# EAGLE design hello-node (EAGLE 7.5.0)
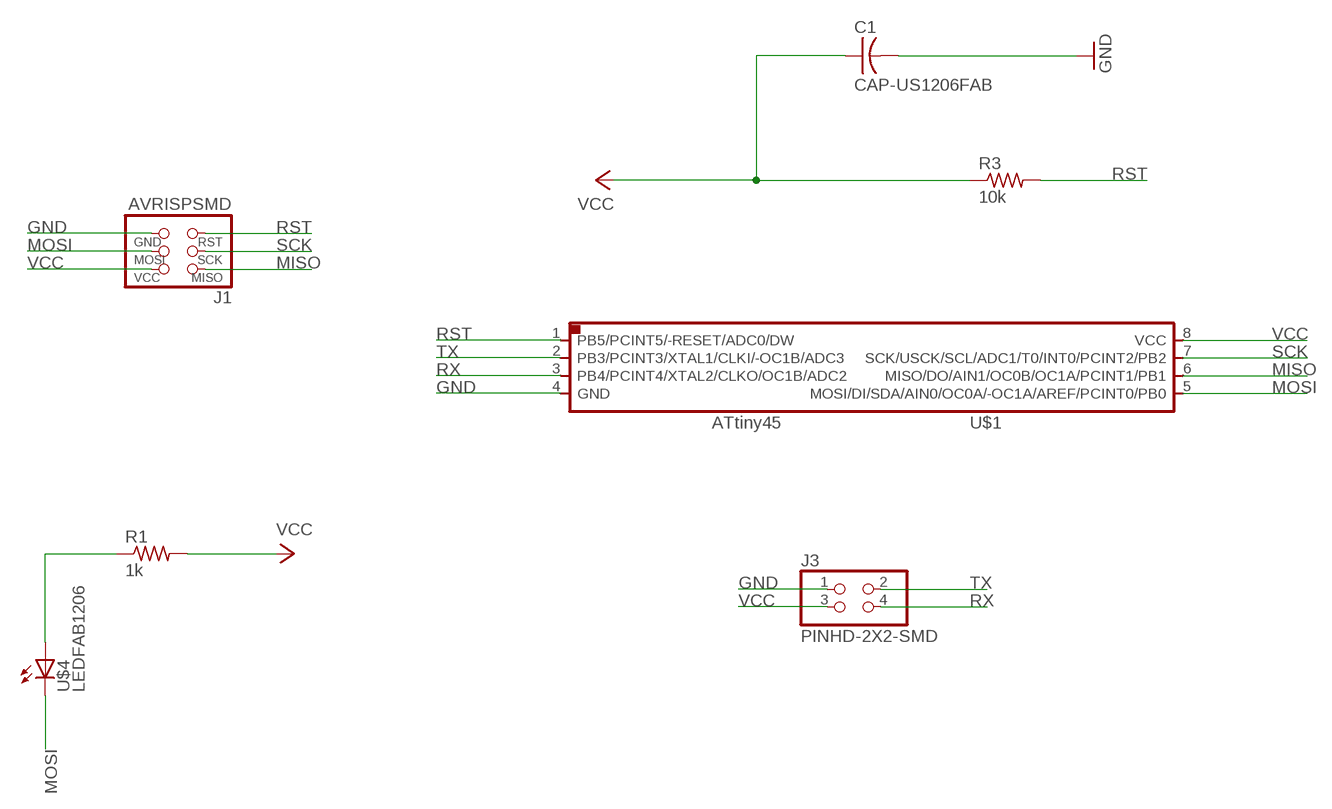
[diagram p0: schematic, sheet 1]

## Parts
C1  CAP-US1206FAB  [C1206FAB]
J1  AVRISPSMD  [2X03SMD]
J3  PINHD-2X2-SMD  [2X02SMD]
R1  1k  RES-US1206FAB  [R1206FAB]
R3  10k  RES-US1206FAB  [R1206FAB]
U$1  ATTINY45SI  [SOIC8]
U$4  LEDFAB1206  [LED1206FAB]

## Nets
GND: C1.2 J1.6(GND) J3.1 U$1.4(GND)
MISO: J1.1(MISO) U$1.6(MISO/DO/AIN1/OC0B/OC1A/PCINT1/PB1)
MOSI: J1.4(MOSI) U$1.5(MOSI/DI/SDA/AIN0/OC0A/-OC1A/AREF/PCINT0/PB0) U$4.2(C)
N$1: R1.1 U$4.1(A)
RST: J1.5(RST) R3.2 U$1.1(PB5/PCINT5/-RESET/ADC0/DW)
RX: J3.4 U$1.3(PB4/PCINT4/XTAL2/CLKO/OC1B/ADC2)
SCK: J1.3(SCK) U$1.7(SCK/USCK/SCL/ADC1/T0/INT0/PCINT2/PB2)
TX: J3.2 U$1.2(PB3/PCINT3/XTAL1/CLKI/-OC1B/ADC3)
VCC: C1.1 J1.2(VCC) J3.3 R1.2 R3.1 U$1.8(VCC)

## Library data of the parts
C1 = 01-fab:CAP-US
J1 = 01-fab:AVRISP
J3 = 01-fab:PINHD-2X2-SMD
R1 R3 = 01-fab:RES-US: Resistor (US Symbol)
U$1 = 01-fab:ATTINY45
U$4 = 01-fab:LED: LED

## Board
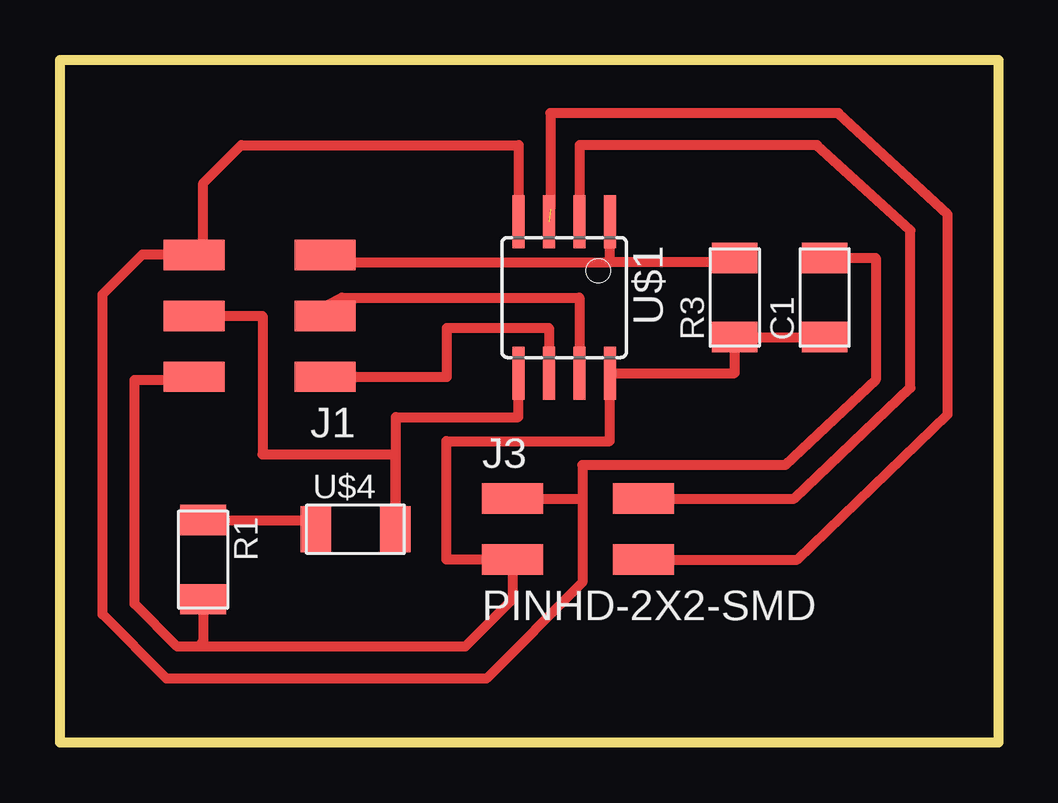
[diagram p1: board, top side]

Size 39.1 x 28.44 mm. Coordinates in mm from the lower left corner, seen from the top.
Outline: 0,0 39.1,0 39.1,28.44 0,28.44 0,0
Copper layers (1*16): Top 0.035mm / dielectric 1.5mm / Bottom 0.035mm
Design rules "default *": minimum track width 10mil, minimum drill 24mil, track to track 16mil, track to pad 16mil, pad to pad 16mil, via to via 16mil, smd to smd 16mil, copper to edge 40mil, drill to drill 8mil, minimum pad ring 10mil, minimum via ring 8mil, stop-mask expansion 4mil, vias tented up to drill 0mil, thermal gap 10mil
Milling: 4 lines

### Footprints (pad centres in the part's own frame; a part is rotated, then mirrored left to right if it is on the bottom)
C1206FAB = smd 1.27 x 1.905: 1 -1.651,0; 2 1.651,0
2X03SMD = smd 2.54 x 1.27: 1 -2.54,2.54; 2 2.92,2.54; 3 -2.54,0; 4 2.92,0; 5 -2.54,-2.54; 6 2.92,-2.54
2X02SMD = smd 2.54 x 1.27: 1 -2.54,1.27; 2 2.92,1.27; 3 -2.54,-1.27; 4 2.92,-1.27
R1206FAB = smd 1.27 x 1.905: 1 -1.651,0; 2 1.651,0
SOIC8 = smd 0.5 x 2.2: 1 -1.905,-3.154; 2 -0.645,-3.154; 3 0.625,-3.154; 4 1.895,-3.154; 5 1.905,3.154; 6 0.635,3.154; 7 -0.635,3.154; 8 -1.905,3.154
LED1206FAB = smd 1.27 x 1.905: 1 -1.651,0; 2 1.651,0

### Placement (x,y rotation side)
C1  31.88,18.54 90 top
J1  8.51,17.78 180 top
J3  21.4,8.89 0 top
R1  5.97,7.62 270 top
R3  28.13,18.54 90 top
U$1  21.02,18.54 180 top
U$4  12.32,8.89 0 top

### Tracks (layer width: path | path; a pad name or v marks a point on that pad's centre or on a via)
GND
  Top 0.406: J1.6 5.97,20.32 5.97,23.3 7.56,24.89 19.12,24.89 U$1.4 | J3.1 21.78,10.16 | 21.78,10.16 21.78,6.67 17.78,2.67 4.45,2.67 1.78,5.33 1.78,18.67 3.44,20.34 5.57,20.34 J1.6 | 5.59,20.34 J1.6 | C1.2 34,20.19 34,15.11 30.23,11.56 21.78,11.56 21.78,10.16
MISO
  Top 0.406: J1.1 16.13,15.24 16.13,17.27 20.38,17.27 U$1.6
MOSI
  Top 0.406: J1.4 8.45,17.78 8.45,12 13.97,12 U$4.2 14,8.89 14,13.56 19.11,13.56 U$1.5
N$1
  Top 0.406: R1.1 10.67,9.27 U$4.1
RST
  Top 0.406: J1.5 11.11,20.32 11.11,20 22.92,20 | R3.2 28,20.19 28,20 22.92,20 | 22.92,20 U$1.1
RX  (1 unrouted)
  Top 0.406: J3.4 30.73,7.62 37.01,13.67 37.01,22 32.45,26.23 20.45,26.23 20.45,22.23
SCK
  Top 0.406: J1.3 10.75,18 11.75,18.54 21.65,18.54 U$1.7
TX
  Top 0.406: J3.2 30.61,10.16 35.45,14.78 35.45,21.34 31.56,24.89 21.66,24.89 U$1.2
VCC
  Top 0.406: C1.1 R3.1 28.13,15.39 U$1.8 22.92,12.56 16.11,12.56 16.11,7.62 J3.3 18.86,5.97 16.89,4 5.78,4 | 5.78,4 4.89,4 3.11,5.78 3.11,15.11 5.59,15.11 J1.2 | R1.2 5.97,4.19 5.78,4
